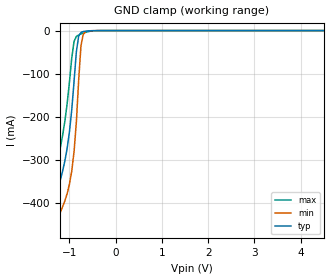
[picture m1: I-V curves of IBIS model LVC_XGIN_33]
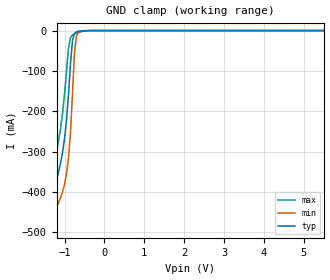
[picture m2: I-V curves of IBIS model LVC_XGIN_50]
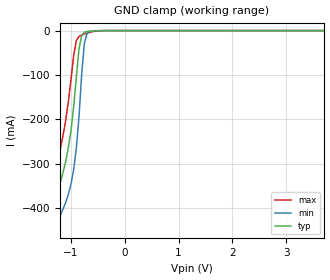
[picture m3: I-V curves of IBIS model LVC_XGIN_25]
| Philips Semiconductors Inc.
| Logic Products Group
| IBIS model of 74LVC1G08
| 3.3V SINGLE 2-INPUT AND GATE
|[Packages]:
|[Package1]: SOT353 (SC88A) 5-pin Package ;
|[Package2]: SOT753 (SC74A) 5-pin Package ;
[IBIS Ver]   3.2
[File Name]   lvc1g08.ibs
[File Rev]   1.1
[Date]   25-Jul-2003
[Source]   File created from simulations by LPG
   Philips Semiconductors Nijmegen
[Notes]   V1.1   Ibis model.
| Revision History
| Version Date   Author/ Description
|   Editor
| 1.0   January 2002 RM   Initial Version
| 1.1   July   2003 RM   Updated Version
| Remarks:
| 1. The Power Clamp curves have been omitted since there is no power clamp
|   diode.
| 2. Non-monotonic sections below 0V in pulldown and pullup curves have been
|   removed (if any).
[Disclaimer]
   (C) Copyright 2003 Philips Semiconductors
   All rights reserved
   Philips Semiconductors warrants and represents that the IBIS model
   identified herein is owned by Philips Semiconductors (PHILIPS). The
   model provided is not warranted as fully representing all of the
   operating characteristics and specifications of the semiconductor
   products to which the model relates.  Moreover, unless there is a
   signed, written agreement to the contrary, this IBIS model is
   furnished on an "as is" basis without support or warranty of any
   kind, either expressed or implied, regarding the use thereof, and
   PHILIPS specifically disclaims all implied warranties of
   merchantability and fitness of the model for any purpose.
   PHILIPS does not assume any liability arising out of the application
   or use of this IBIS model including infringement of patents and
   copyrights, nor does PHILIPS convey any license under its patents and
   copyrights or the rights of others.
   PHILIPS provides IBIS models as a service to our customers. You and
   your company shall not distribute, convey, sell, or give these models
   to anyone else without receiving prior written permission from
   PHILIPS.
   PHILIPS reserves the right to make changes without notice to these
   IBIS models to improve reliability, function, or design.
   Please be aware that your receipt and subsequent use of the IBIS
   information provided shall serve as acceptance of the terms and
   conditions of this agreement.  If you do not accept these terms,
   you should return or destroy the IBIS models and any other
   accompanying information immediately.
|   Info for  SOT353 (SC88A) 5-pin Package
[Component]   74LVC1G08_1
[Manufacturer]   Philips Semiconductors Inc.
[package]
|   typ   min   max
R_pkg   966.6e-6   950e-6   979e-6
L_pkg   390.8e-12   388e-12   393e-12
C_pkg   69.2e-15   46e-15   127e-15
[Pin] signal_name   model_name   R_pin   L_pin   C_pin
   1   B   lvc_xgin   967e-6   393e-12   46e-15
   2   A   lvc_xgin   950e-6   388e-12   61e-15
   3   GND   GND   967e-6   392e-12   127e-15
   4   Y   lvc_xgoutn   979e-6   391e-12   59e-15
   5   VCC   POWER   970e-6   390e-12   49e-15
|   Info for  SOT753 (SC74A) 5-pin Package
[Component]   74LVC1G08_2
[Manufacturer]   Philips Semiconductors Inc.
[package]
|   typ   min   max
R_pkg   7.0863E-02   5.8319E-02   8.4334E-02
L_pkg   8.780E-10   7.160E-10   1.003E-09
C_pkg   8.44E-14   5.30E-14   1.63E-13
[Pin] signal_name   model_name   R_pin   L_pin   C_pin
   1   B   lvc_xgin 8.43E-02  9.97E-10  7.40E-14
   2   A   lvc_xgin 5.83E-02  7.16E-10  5.30E-14
   3   GND   GND 7.08E-02 1.003E-09  1.63E-13
   4   Y   lvc_xgoutn 7.04E-02   8.2E-10  6.30E-14
   5   VCC   POWER 7.04E-02  8.54E-10  6.90E-14
[Model Selector]   lvc_xgin
| Remark: If your software does not support the Model Selector
|   Please comment out the lines of the Model Selector, which
|   contain the name of the Model, except the one you want to use.
LVC_XGIN_33   3.3V-Vcc input model
LVC_XGIN_50   5.0V-Vcc input model
LVC_XGIN_25   2.5V-Vcc input model
LVC_XGIN_18   1.8V-Vcc input model
[Model Selector]   lvc_xgoutn
| Remark: If your software does not support the Model Selector
|   Please comment out the lines of the Model Selector, which
|   contain the name of the Model, except the one you want to use.
LVC_XGOUTN_33   3.3V-Vcc output model (non-inverting)
LVC_XGOUTN_50   5.0V-Vcc output model (non-inverting)
LVC_XGOUTN_25   2.5V-Vcc output model (non-inverting)
LVC_XGOUTN_18   1.8V-Vcc output model (non-inverting)
| Models and submodels in the file (8): LVC_XGIN_33 (Input), LVC_XGIN_50 (Input), LVC_XGIN_25 (Input), LVC_XGIN_18 (Input), LVC_XGOUTN_33 (Output), LVC_XGOUTN_50 (Output), LVC_XGOUTN_25 (Output), LVC_XGOUTN_18 (Output)
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|   Model LVC_XGIN_33
[Model]   LVC_XGIN_33
Model_type   Input
Vinl =   0.8V
Vinh =   2.0V
C_comp   2.96pF   2.12pF   3.91pF
[Model Spec]
| Note: The input and output voltage ratings may be exceeded if the input and
|   output current ratings are observed (please refer to the data sheet)
|   Subparameter   typ   min   max
| Thresholds
Vinh   2.0   2.0   2.0
Vinl   0.8   0.8   0.8
| Overshoot
S_overshoot_high   6.5   6.5   6.5   | Static overshoot
S_overshoot_low   -0.5   -0.5   -0.5
D_overshoot_high   7.2   7.2   7.2   | Dynamic overshoot
D_overshoot_low   -0.95   -0.9   -1.0
D_overshoot_time   3n   3n   3n
|Ambient temperature:   25   85   -40
[Temperature Range]   50   105   -10
[Voltage Range]   3.3V   3.0V   3.6V
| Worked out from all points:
|   GND clamp passes 1 mA (typ) near -0.61 V on its own axis
|Process Range   nominal   slow   fast
[GND_clamp]
| voltage   I(typ)   I(min)   I(max)
-5.5V     -4.562A    -4.619A    -4.506A
-1.45V    -549.4mA   -615.4mA   -482.8mA
-1.4V     -502.2mA   -568.5mA   -435.4mA
-1.35V    -455.9mA   -522.5mA   -388.7mA
-1.3V     -411.6mA   -478.9mA   -343.8mA
-1.1V     -304.2mA   -396.4mA   -212.1mA
-950mV    -185.2mA   -327mA     -64.69mA
-850mV    -49.8mA    -213.4mA   -13.79mA
-750mV    -4.324mA   -35.6mA    -7.884mA
-700mV    -2.27mA    -8.526mA   -5.841mA
-550mV    -593.6uA   -425.2uA   -1.597mA
5.5V      375.8pA    2.471nA    52.76pA
|   Model LVC_XGIN_50
[Model]   LVC_XGIN_50
Model_type   Input
Vinl =   1.5V
Vinh =   3.5V
C_comp   2.89pF   1.97pF   3.94pF
[Model Spec]
| Note: The input and output voltage ratings may be exceeded if the input and
|   output current ratings are observed (please refer to the data sheet)
|   Subparameter   typ   min   max
| Thresholds
Vinh   3.5   3.15   3.85
Vinl   1.5   1.35   1.65
| Overshoot
S_overshoot_high   6.5   6.5   6.5   | Static overshoot
S_overshoot_low   -0.5   -0.5   -0.5
D_overshoot_high   11.0   11.0   11.0   | Dynamic overshoot
D_overshoot_low   -0.95   -0.9   -1.0
D_overshoot_time   3n   3n   3n
|Ambient temperature:   25   85   -40
[Temperature Range]   50   105   -10
[Voltage Range]   5.0V   4.5V   5.5V
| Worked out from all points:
|   GND clamp passes 1 mA (typ) near -0.59 V on its own axis
|Process Range   nominal   slow   fast
[GND_clamp]
| voltage   I(typ)   I(min)   I(max)
-5.5V     -4.585A    -4.637A    -4.534A
-1.45V    -567.8mA   -628.4mA   -505.9mA
-1.4V     -520.6mA   -581.5mA   -458.5mA
-1.3V     -430.1mA   -491.9mA   -367mA
-1.2V     -369.6mA   -437.9mA   -299.9mA
-1.05V    -303mA     -399.7mA   -205.6mA
-950mV    -222.3mA   -354.8mA   -100.4mA
-850mV    -82.04mA   -253.9mA   -17.37mA
-800mV    -24.94mA   -156mA     -10.72mA
-750mV    -6.792mA   -54.58mA   -8.095mA
-700mV    -2.837mA   -13.44mA   -6.14mA
5.5V      1.794nA    5.479nA    963.8pA
|   Model LVC_XGIN_25
[Model]   LVC_XGIN_25
Model_type   Input
Vinl =   0.7V
Vinh =   1.7V
C_comp   3.01pF   2.23pF   3.90pF
[Model Spec]
| Note: The input and output voltage ratings may be exceeded if the input and
|   output current ratings are observed (please refer to the data sheet)
|   Subparameter   typ   min   max
| Thresholds
Vinh   1.7   1.7   1.7
Vinl   0.7   0.7   0.7
| Overshoot
S_overshoot_high   6.5   6.5   6.5   | Static overshoot
S_overshoot_low   -0.5   -0.5   -0.5
D_overshoot_high   7.2   7.2   7.2   | Dynamic overshoot
D_overshoot_low   -0.95   -0.9   -1.0
D_overshoot_time   3n   3n   3n
|Ambient temperature:   25   85   -40
[Temperature Range]   30   90   -35
[Voltage Range]   2.5V   2.3V   2.7V
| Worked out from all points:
|   GND clamp passes 1 mA (typ) near -0.61 V on its own axis
|Process Range   nominal   slow   fast
[GND_clamp]
| voltage   I(typ)   I(min)   I(max)
-5.5V     -4.553A    -4.61A     -4.497A
-1.45V    -543.2mA   -609mA     -477mA
-1.4V     -496.1mA   -562.1mA   -429.6mA
-1.35V    -449.7mA   -516.1mA   -382.9mA
-1.25V    -367.8mA   -436.8mA   -298.4mA
-1.1V     -295.9mA   -387.6mA   -204.4mA
-950mV    -173.1mA   -313.3mA   -57.16mA
-850mV    -41.37mA   -194.3mA   -13.46mA
-750mV    -3.847mA   -28.54mA   -7.836mA
-700mV    -2.146mA   -6.789mA   -5.759mA
-550mV    -554.2uA   -385.7uA   -1.497mA
5.5V      211.8pA    1.646nA    21.33pA
